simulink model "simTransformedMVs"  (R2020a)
settings: Solver=ode15s  StartTime=0.0  StopTime=tsim  RelTol=1e-3
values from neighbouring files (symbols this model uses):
  dF = 1;0*F0    [TransformedMVs.m]
  dT = 1;0*T0    [TransformedMVs.m]
  dT1 = 0.15*T10    (= 3)    [TransformedMVs.m]
  dT2 = 0.1*T20    (= 5)    [TransformedMVs.m]
  F0 = 10    [TransformedMVs.m]
  Kc = 1/k.T*tau.T/(tauC.T+theta)    [TransformedMVs.m]    (also in Main.m = 1/k*tau/(tauC+theta); runTransf.m = 1/kM(i)*tau(i)/(tauCM(i)+theta(i)); runTransfOL.m = 1/kM(i)*tau(i)/(tauCM(i)+theta(i)))
  KI = 1/k.F/(tauC.F+theta)    [TransformedMVs.m]    (also in Main.m = Kp/tauIv; Main_OL.m = 1; runTransf.m = 1/kS(i)*1/tauCS(i); runTransfOL.m = 1/kS(i)*1/tauCS(i))
  p = [m; tau0]    [TransformedMVs.m]    (also in Main.m = [N, Fc0, rhoc, rhoh,U,A,cpc,cph]; Main_OL.m = [N, Fc0, rhoc, rhoh,U,A,cpc,cph]; runTestCalcBlk.m = [N, Fc0, rhoc, rhoh,U,A,cpc,cph]; NonlinearMap.m = [U;A;Fc(i);Fh;cpc;cph;Tcin;Thin])
  T0 = 35    [hmeas.m]    (also in TransformedMVs.m; H2P_Turbine_driven.m = param(9); runTD.m = 318; H2P_Boiler_driven.m = param(9))
  T10 = 20    [TransformedMVs.m]
  T20 = 50    [TransformedMVs.m]
  tauI = min(tau.T,4*(tauC.T+theta))    [TransformedMVs.m]    (also in Main.m = min(tau,4*(tauC+theta)); runTransf.m = min(tau(i), 4*(tauCM(i)+theta(i))); runTransfOL.m = min(tau(i), 4*(tauCM(i)+theta(i))))
  tstep_d1 = 50    [TransformedMVs.m]
  tstep_d2 = 100    [TransformedMVs.m]
  tstep_F = 200    [TransformedMVs.m]
  tstep_T = 150    [TransformedMVs.m]
  v1_0 = F10+F20    (= 10)    [TransformedMVs.m]
  v2_0 = tau0/m*(F10*T10+F20*T20)+(1-tau0/taur0)*T0    (= 35)    [TransformedMVs.m]
undefined symbols (not defined in the file or in its folder): CalcBlock, shower

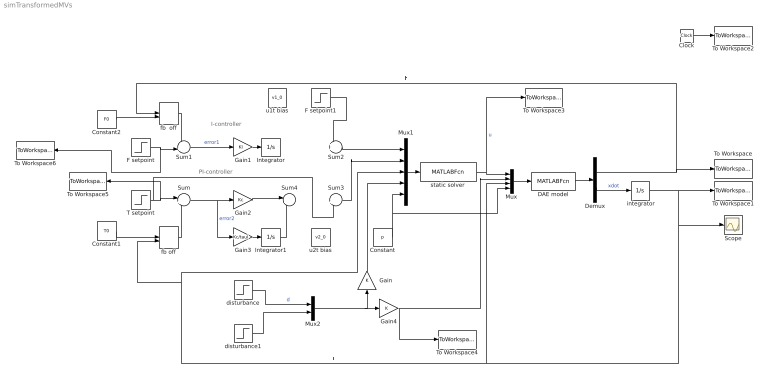
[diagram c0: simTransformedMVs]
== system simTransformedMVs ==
  note: PI-controller
  note: I-controller
  " integrator" : Integrator  InitialCondition=T0
  Clock : Clock
  Constant : Constant  Value=p
  Constant1 : Constant  Value=T0
  Constant2 : Constant  Value=F0
  DAE model : MATLABFcn  MATLABFcn=shower(u(1:2), u(3:4),u(5),u(6:7))  OutputDimensions=2
  Demux : Demux  Outputs=2
  F setpoint : Step  Time=tstep_F  Before=F0  After=F0+dF  SampleTime=0
  F setpoint1 : Step  Time=tstep_F  Before=F0  After=F0+dF  SampleTime=0
  Gain : Gain
  Gain1 : Gain  Gain=KI  Multiplication=Matrix(K*u)
  Gain2 : Gain  Gain=Kc  Multiplication=Matrix(K*u)
  Gain3 : Gain  Gain=Kc/tauI  Multiplication=Matrix(K*u)
  Gain4 : Gain
  Integrator : Integrator
  Integrator1 : Integrator
  Mux : Mux
  Mux1 : Mux  Inputs=5
  Mux2 : Mux  Inputs=2
  Scope : Scope
  Sum : Sum  Inputs=|+-
  Sum1 : Sum  Inputs=-+|
  Sum2 : Sum  Inputs=++|
  Sum3 : Sum  Inputs=|++
  Sum4 : Sum  Inputs=|++
  T setpoint : Step  Time=tstep_T  Before=T0  After=T0+dT  SampleTime=0
  To Workspace : ToWorkspace  VariableName=F  SampleTime=-1
  To Workspace1 : ToWorkspace  VariableName=T  SampleTime=-1
  To Workspace2 : ToWorkspace  VariableName=time  SampleTime=-1
  To Workspace3 : ToWorkspace  VariableName=u  SampleTime=-1
  To Workspace4 : ToWorkspace  VariableName=d  SampleTime=-1
  To Workspace5 : ToWorkspace  VariableName=Tsp  SampleTime=-1
  To Workspace6 : ToWorkspace  VariableName=Fsp  SampleTime=-1
  disturbance : Step  Time=tstep_d1  Before=T10  After=T10+dT1  SampleTime=0
  disturbance1 : Step  Time=tstep_d2  Before=T20  After=T20+dT2  SampleTime=0
  fb  off : ManualSwitch
  fb off : ManualSwitch  CurrentSetting=0
  static solver : MATLABFcn  MATLABFcn=CalcBlock(u(1:2),u(3),u(4:5),u(6:7))  OutputDimensions=2
  u1t bias : Constant  Value=v1_0
  u2t bias : Constant  Value=v2_0
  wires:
  DAE model/1 -> Demux/1
  Demux/1 -> fb  off/1, To Workspace/1  "F"
  " integrator"/1 -> To Workspace1/1, Scope/1, Mux/3, Mux1/3, fb off/2  "T"
  Mux/1 -> DAE model/1
  Clock/1 -> To Workspace2/1
  Sum/1 -> Gain3/1, Gain2/1  "error2"
  T setpoint/1 -> Sum3/2, To Workspace5/1, Sum/1
  Sum1/1 -> Gain1/1  "error1"
  F setpoint/1 -> To Workspace6/1, Sum1/2
  static solver/1 -> To Workspace3/1, Mux/1  "u"
  Gain1/1 -> Integrator/1
  Sum4/1 -> ?  "v2"
  u1t bias/1 -> ?
  u2t bias/1 -> ?
  Mux1/1 -> static solver/1
  Sum2/1 -> Mux1/1
  Sum3/1 -> Mux1/2
  Demux/2 -> " integrator"/1  "xdot"
  disturbance/1 -> Mux2/1  "d"
  Mux2/1 -> Gain/1, Gain4/1
  Integrator/1 -> ?  "v1"
  Gain3/1 -> Integrator1/1
  Gain2/1 -> Sum4/1
  Integrator1/1 -> Sum4/2
  Constant/1 -> Mux1/5, Mux/4
  disturbance1/1 -> Mux2/2
  Gain4/1 -> Mux/2, To Workspace4/1
  Constant2/1 -> fb  off/2
  fb  off/1 -> Sum1/1
  fb off/1 -> Sum/2
  Constant1/1 -> fb off/1
  Gain/1 -> Mux1/4
  F setpoint1/1 -> Sum2/1
